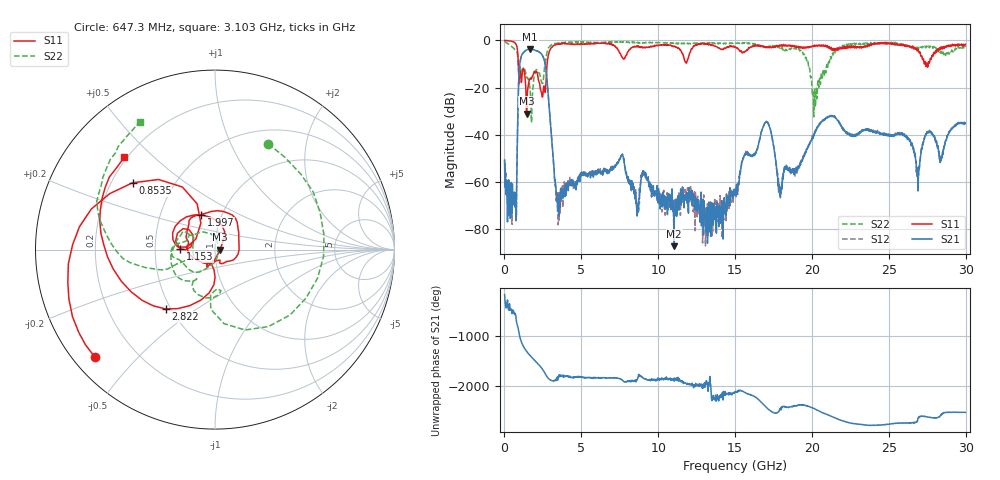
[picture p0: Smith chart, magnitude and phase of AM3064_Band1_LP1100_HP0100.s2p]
# Hz S DB R 50.0
!freq dBS11 angS11 dBS21 angS21 dBS12 angS12 dBS22 angS22
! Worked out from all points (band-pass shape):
!   1600 points, 10 MHz to 29.98 GHz, reference 50 ohm
!   highest |S21| = -3.74 dB at 1.659 GHz (marker M1); lowest = -87.1 dB at 11.03 GHz (marker M2)
!   |S21| within 3 dB of the highest: 1.095 GHz to 2.499 GHz (1.404 GHz wide, 78.1 % of centre)
!   lowest |S11| = -31.0 dB at 1.435 GHz (marker M3), VSWR 1.06, Z = 52.9 - j0.0523 ohm
!   |S11| at or under -10 dB: 902.2 MHz to 2.775 GHz (1.872 GHz wide, 102 % of centre); 27.39213 GHz to 27.45943 GHz (67.29 MHz wide, 0.245 % of centre); 27.48984 GHz to 27.56386 GHz (74.02 MHz wide, 0.269 % of centre)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
!   |S22| runs from -34.8 to -0.4 dB; largest |S21 - S12| = 0.0084
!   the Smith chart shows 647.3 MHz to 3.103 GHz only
!   S11 on the Smith chart (normalised r, x): 647.3 MHz: 0.06, -0.38; 853.5 MHz: 0.29, +0.33; 1.153 GHz: 0.68, +0.01; 1.997 GHz: 0.80, +0.32; 2.822 GHz: 0.47, -0.38; 3.103 GHz: 0.19, +0.41
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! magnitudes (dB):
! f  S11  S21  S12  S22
! 10 MHz  0.0  -51.0  -50.2  -0.4
! 647.3 MHz  -0.9  -64.2  -67.6  -3.6
! 853.5 MHz  -4.6  -37.3  -37.3  -6.4
! 1.153 GHz  -14.3  -5.9  -5.9  -13.4
! 1.435 GHz  -31.0  -4.1  -4.0  -15.9
! 1.659 GHz  -16.3  -3.7  -3.7  -20.5
! 1.997 GHz  -13.5  -4.2  -4.1  -14.2
! 2.822 GHz  -7.3  -21.0  -20.8  -3.9
! 3.103 GHz  -2.8  -44.0  -44.5  -1.7
! 3.496 GHz  -1.6  -67.1  -78.1  -1.1
! 5.015 GHz  -1.6  -55.8  -57.0  -0.7
! 7.62 GHz  -6.9  -48.5  -48.7  -0.7
! 8.632 GHz  -2.7  -74.4  -70.4  -1.0
! 10 GHz  -2.1  -68.7  -64.8  -1.0
! 11.03 GHz  -2.5  -87.1  -71.4  -1.1
! 15 GHz  -3.0  -65.1  -63.7  -1.3
! 16.99 GHz  -3.0  -34.6  -34.6  -2.7
! 17.93 GHz  -2.0  -63.9  -61.5  -2.7
! 19.99 GHz  -2.8  -41.8  -41.7  -18.1
! 25 GHz  -1.1  -40.3  -40.5  -1.1
! 26.89 GHz  -4.1  -57.1  -57.2  -3.3
! 29.98 GHz  -1.7  -35.1  -35.1  -2.9
